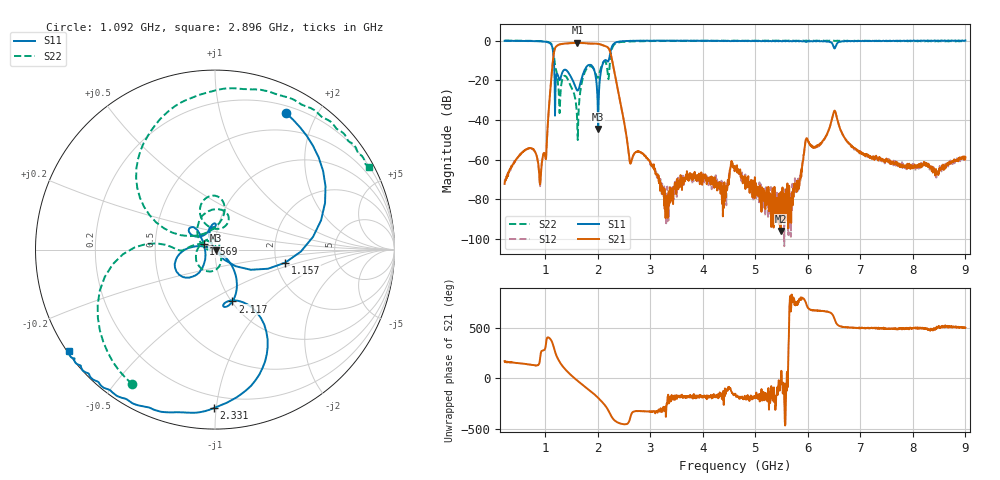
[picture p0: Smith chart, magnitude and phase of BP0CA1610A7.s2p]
!Agilent Technologies,E8358A,US41080443,A.07.50.56
!Agilent E8358A: A.07.50.56
!Date: Tuesday, April 11, 2017 15:45:42
!Correction: S11(Full 2 Port(1,2))
!S21(Full 2 Port(1,2))
!S12(Full 2 Port(1,2))
!S22(Full 2 Port(1,2))
!S2P File: Measurements: S11, S21, S12, S22:
# Hz S  dB  R 50
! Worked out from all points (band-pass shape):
!   1601 points, 225 MHz to 9 GHz, reference 50 ohm
!   highest |S21| = -1.10 dB at 1.613 GHz (marker M1); lowest = -95.8 dB at 5.479 GHz (marker M2)
!   |S21| within 3 dB of the highest: 1.181 GHz to 2.211 GHz (1.03 GHz wide, 60.7 % of centre)
!   lowest |S11| = -44.5 dB at 2.007 GHz (marker M3), VSWR 1.01, Z = 50.5 - j0.359 ohm
!   |S11| at or under -10 dB: 1.163 GHz to 2.128 GHz (965 MHz wide, 58.7 % of centre); 2.164 GHz to 2.206 GHz (41.5 MHz wide, 1.9 % of centre)
!   |S22| runs from -50.0 to 0.0 dB; largest |S21 - S12| = 0.0095
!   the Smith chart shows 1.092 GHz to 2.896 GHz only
!   S11 on the Smith chart (normalised r, x): 1.092 GHz: 0.28, +1.61; 1.157 GHz: 2.24, -0.39; 1.569 GHz: 0.88, +0.06; 2.117 GHz: 1.01, -0.64; 2.331 GHz: 0.12, -0.98; 2.896 GHz: 0.01, -0.31
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2.25e8  -0.09 169.0  -72.17 171.1  -71.32 163.8  0.00 -10.7
6.747188e8  -0.21 141.8  -54.31 139.9  -54.39 139.9  -0.07 -39.0
9.105469e8  -0.39 115.5  -70.25 -115.7  -69.31 -113.6  -0.24 -67.4
1.091531e9  -1.34 62.4  -26.11 31.7  -26.16 32.0  -1.11 -121.6
1.157344e9  -7.99 -10.5  -7.22 -45.4  -7.28 -45.3  -5.80 -177.2
1.272516e9  -19.93 123.3  -1.86 164.2  -1.96 164.2  -36.50 31.1
1.393172e9  -14.77 136.9  -1.42 82.8  -1.51 82.8  -18.14 -140.3
1.568672e9  -22.95 153.9  -1.12 -3.0  -1.20 -2.9  -29.04 47.3
1.612547e9  -25.14 -173.9  -1.10 -22.1  -1.19 -22.0  -44.71 -17.3
1.689328e9  -19.28 -126.3  -1.15 -54.6  -1.23 -54.6  -21.85 159.2
2.007422e9  -44.47 -36.4  -1.60 168.1  -1.69 168.2  -18.51 95.0
2.117109e9  -10.33 -71.4  -2.53 107.0  -2.60 107.2  -10.51 96.5
2.331e9  -1.08 -90.4  -18.10 -58.5  -18.11 -58.7  -1.52 103.5
2.616188e9  -0.11 -130.4  -61.82 -29.7  -61.76 -29.8  -0.43 50.5
2.895891e9  -0.08 -145.1  -58.05 36.4  -58.05 35.7  -0.23 28.1
3.153656e9  -0.07 -153.5  -67.79 45.0  -69.09 27.6  -0.17 13.6
4.6125e9  -0.13 178.6  -65.34 -160.1  -64.34 -175.2  -0.08 -28.3
5.479031e9  -0.18 160.4  -95.84 -28.1  -89.44 -179.8  -0.11 -39.0
6.076828e9  -0.30 147.8  -52.80 -44.8  -53.45 -45.1  -0.07 -45.0
6.510094e9  -3.95 143.6  -35.25 -135.8  -35.45 -136.3  -0.11 -51.1
7.541156e9  -0.19 131.6  -61.34 134.1  -59.57 129.5  -0.12 -67.0
9e9  0.08 123.1  -58.82 140.9  -58.84 144.4  -0.34 -96.8
